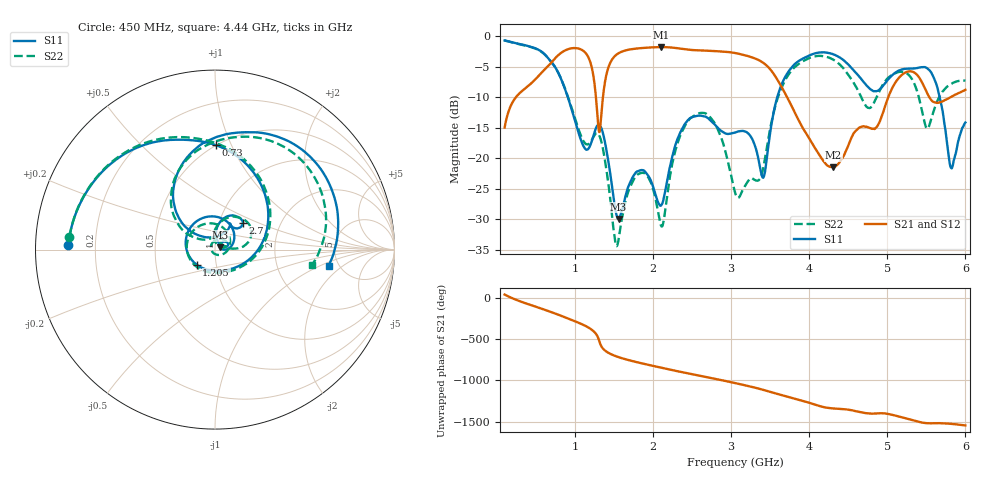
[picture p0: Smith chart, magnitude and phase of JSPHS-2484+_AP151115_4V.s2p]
!Mini-Circuits Laboratory
!S-Parameters
!Run/Lot/Date Code:MF33450/NA/1551
!Fixture/SN/Due: 90-4-20-21/70546/03/17/16
!Connection:PORT<IN> - pin<1>; PORT<OUT> - pin<7>;PORT<BIAS> - pin<4>;
!Tested With:PORT EXTENTION
!Network Analyzer:AG E5071C/74883/05/12/16
!Created: 01-07-2016 at 14:09:31
!MODEL: JSPHS-2484+
!S/N: V=4V
# MHZ S DB R 50
!Frequency  S11 dB  S11 DEG  S21 dB  S21 DEG  S12 dB  S12 DEG  S22 dB  S22 DEG
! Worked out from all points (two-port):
!   1181 points, 100 MHz to 6 GHz, reference 50 ohm
!   highest |S21| = -1.74 dB at 2.1 GHz (marker M1); lowest = -21.4 dB at 4.31 GHz (marker M2)
!   |S21| within 3 dB of the highest: 665 MHz to 1.209 GHz (544.4 MHz wide, 58.1 % of centre); 1.438 GHz to 3.453 GHz (2.014 GHz wide, 82.4 % of centre)
!   lowest |S11| = -29.9 dB at 1.56 GHz (marker M3), VSWR 1.07, Z = 52.9 + j1.46 ohm
!   |S11| at or under -10 dB: 910.4 MHz to 3.59 GHz (2.679 GHz wide, 119 % of centre); 5.671 GHz to end of sweep
!   |S22| runs from -34.4 to -0.7 dB; largest |S21 - S12| = 0.0034
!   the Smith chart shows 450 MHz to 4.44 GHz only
!   S11 on the Smith chart (normalised r, x): 450 MHz: 0.10, +0.02; 730 MHz: 0.50, +0.88; 1.205 GHz: 0.80, -0.14; 2.7 GHz: 1.30, +0.40; 4.44 GHz: 4.15, -1.25
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100  -0.66 -52.5  -14.93 37.1  -14.93 37.1  -0.65 -52.6
450  -1.76 178.1  -7.57 -94.2  -7.56 -94.2  -1.78 174.9
730  -4.70 89.6  -3.81 174.7  -3.81 174.7  -4.72 85.9
930  -10.77 15.3  -2.01 101.2  -2.01 101.2  -10.60 13.3
1085  -17.25 -53.2  -2.17 41.0  -2.17 41.0  -16.52 -52.2
1205  -17.57 -140.5  -4.54 -20.3  -4.53 -20.3  -17.22 -130.0
1330  -14.79 85.4  -14.09 148.6  -14.09 148.6  -16.84 90.6
1560  -29.92 25.6  -2.74 1.1  -2.74 1.0  -33.21 171.0
1810  -22.05 30.2  -1.95 -63.2  -1.95 -63.3  -22.58 47.6
2070  -27.32 32.3  -1.75 -118.8  -1.75 -118.8  -29.14 19.4
2100  -27.77 49.3  -1.74 -125.0  -1.74 -125.1  -30.96 36.7
2700  -13.36 43.7  -2.34 117.9  -2.34 117.8  -12.85 26.7
3050  -15.76 58.6  -2.71 48.6  -2.71 48.6  -25.58 25.7
3505  -15.33 143.1  -5.45 -58.9  -5.45 -58.9  -14.78 150.6
4035  -2.94 63.6  -17.48 159.2  -17.43 159.1  -3.38 64.4
4310  -2.93 17.0  -21.44 101.4  -21.50 100.7  -3.81 16.5
4440  -3.88 -8.0  -19.61 93.4  -19.62 94.7  -5.25 -9.3
4755  -8.30 -90.4  -14.91 41.4  -14.87 41.8  -11.70 -125.1
5020  -6.91 144.1  -9.70 33.8  -9.69 33.7  -6.68 110.8
5500  -5.13 21.8  -9.01 -75.8  -9.02 -75.8  -15.00 55.1
5815  -21.53 1.2  -9.93 -83.7  -9.93 -83.7  -7.80 73.6
6000  -14.11 36.4  -8.75 -103.4  -8.75 -103.4  -7.25 58.9
